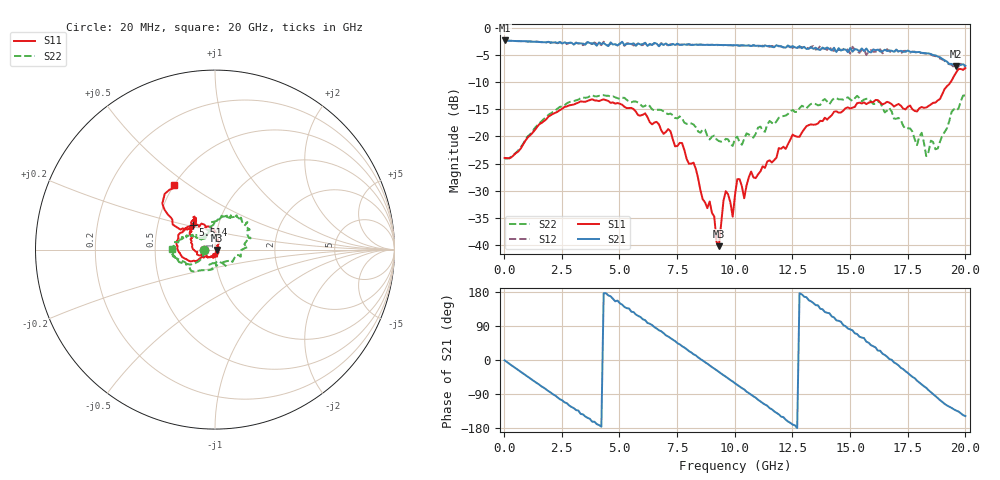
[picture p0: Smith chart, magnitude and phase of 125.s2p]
!Agilent Technologies,N5230A,US43500223,A.07.50.48
!Agilent N5230A: A.07.50.48
!Date: Monday, September 14, 2015 17:31:43
!Correction: S11(Full 2 Port(1,2))
!S21(Full 2 Port(1,2))
!S12(Full 2 Port(1,2))
!S22(Full 2 Port(1,2))
!S2P File: Measurements: S11, S21, S12, S22:
# Hz S  dB  R 50
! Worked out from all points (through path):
!   201 points, 20 MHz to 20 GHz, reference 50 ohm
!   highest |S21| = -2.29 dB at 20 MHz (marker M1); lowest = -7.0 dB at 19.6 GHz (marker M2)
!   group delay of S21, straight-line fit = 120 ps
!   lowest |S11| = -40.2 dB at 9.311 GHz (marker M3), VSWR 1.02, Z = 51 - j0.197 ohm
!   |S11| at or under -10 dB: start of sweep to 19.35 GHz
!   |S22| runs from -24.1 to -12.4 dB; largest |S21 - S12| = 0.085
!   S11 on the Smith chart (normalised r, x): 20 MHz: 0.88, -0.00; 5.514 GHz: 0.75, +0.21; 20 GHz: 0.50, +0.44
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2e7  -23.96 -179.5  -2.29 -0.9  -2.30 -0.9  -24.04 -179.7
1.9181e9  -16.34 -154.5  -2.54 -82.0  -2.56 -82.4  -16.02 -148.1
3.4166e9  -13.59 176.1  -2.86 -143.5  -3.16 -142.8  -12.80 -166.7
4.3157e9  -13.15 158.4  -2.78 176.3  -2.51 178.4  -12.39 179.5
5.5145e9  -14.74 132.3  -2.95 127.6  -2.96 126.9  -13.69 165.1
6.7133e9  -17.78 100.5  -3.37 78.5  -3.23 80.1  -15.08 152.9
8.2118e9  -24.84 75.9  -3.11 15.2  -3.05 15.9  -17.79 146.5
9.3107e9  -40.24 -11.5  -3.12 -31.3  -3.13 -30.9  -20.85 144.6
9.6104e9  -30.10 -68.9  -3.13 -44.1  -3.18 -43.7  -20.44 138.7
9.9101e9  -34.80 -53.8  -3.18 -56.8  -3.21 -56.7  -21.74 129.2
1.001e10  -30.79 -64.3  -3.16 -61.4  -3.17 -61.0  -20.34 129.3
1.08092e10  -27.56 -113.0  -3.14 -95.9  -3.27 -95.0  -20.21 113.2
1.2008e10  -22.28 -154.7  -3.38 -149.3  -3.38 -147.3  -16.34 95.3
1.34066e10  -17.85 170.3  -3.83 150.4  -3.34 149.9  -13.87 72.2
1.43057e10  -15.43 146.7  -3.64 112.4  -4.21 110.2  -12.95 56.2
1.51049e10  -14.68 132.4  -4.37 78.2  -3.45 78.2  -13.44 43.5
1.67033e10  -13.76 121.0  -4.13 2.6  -4.32 2.6  -14.75 4.6
1.79021e10  -15.39 138.0  -4.45 -54.5  -4.62 -53.9  -21.59 -56.7
1.81019e10  -14.57 137.9  -4.57 -64.1  -4.59 -63.5  -19.32 -56.4
1.83017e10  -14.66 140.4  -4.66 -73.3  -4.76 -73.6  -23.63 -75.6
1.96004e10  -8.19 138.9  -7.00 -133.5  -7.23 -131.3  -15.21 -146.7
2e10  -7.39 122.6  -6.97 -148.0  -7.21 -147.6  -12.44 178.9
